(* Logix 5000 AddOnInstructionDefinition export Banner_Q90R2_KD_PD_v4; software revision 33.00 *)

TYPE Banner_Q90R2KD_PDI_0_v4 :   // Process Data for a Q90R2 sensors.
STRUCT
   SSC1_State : SINT;   // 0 = Inactive 1 = Active
   SSC1_Stability : SINT;   // 0 = No target or maginal, 1 = Valid.
   SSC2_State : SINT;   // 0 = Inactive 1 = Active
   SSC2_Stability : SINT;   // 0 = No target or maginal, 1 = Valid.
   SSC1_Distance : DINT;
   SSC1_Beam_Angle : DINT;
   SSC1_Velocity : DINT;
   SSC1_Signal_Strength : DINT;
   SSC2_Distance : DINT;
   SSC2_Beam_Angle : DINT;
   SSC2_Velocity : DINT;
   SSC2_Signal_Strength : DINT;
END_STRUCT
END_TYPE

TYPE Banner_Q90R2KD_PDI_1_v4 :   // Process Data for a Q90R2 sensors.
STRUCT
   SSC1_State : SINT;   // 0 = Inactive, 1 = True.
   SSC1_Stability : SINT;   // 0 = No target or maginal, 1 = Valid.
   SSC2_State : SINT;   // 0 = Inactive, 1 = True.
   SSC2_Stability : SINT;   // 0 = No target or maginal, 1 = Valid.
   SSC1_X : DINT;
   SSC1_Y : DINT;
   SSC1_Velocity : DINT;
   SSC1_Signal_Strength : DINT;
   SSC2_X : DINT;
   SSC2_Y : DINT;
   SSC2_Velocity : DINT;
   SSC2_Signal_Strength : DINT;
END_STRUCT
END_TYPE

TYPE Banner_Q90R2KD_PDI_v4 :   // Process Data for a Q90R2 sensors.
STRUCT
   Set_0 : Banner_Q90R2KD_PDI_0_v4;
   Set_1 : Banner_Q90R2KD_PDI_1_v4;
   PDI_DT : SINT[16];
END_STRUCT
END_TYPE

ADD_ON_INSTRUCTION Banner_Q90R2_KD_PD_v4   (* revision 4.0, vendor Banner Engineering *)
// Take raw process data and convert it to usable values.
VAR_IN_OUT
   PD : Banner_Q90R2KD_PDI_v4; {required}
END_VAR
VAR_INPUT
   PD_Layout : SINT; {required}
   Byte_Swap : BOOL; {required}
END_VAR
VAR
   Temp : SINT[16]; {access None}
END_VAR

ROUTINE Logic   (* ladder *)
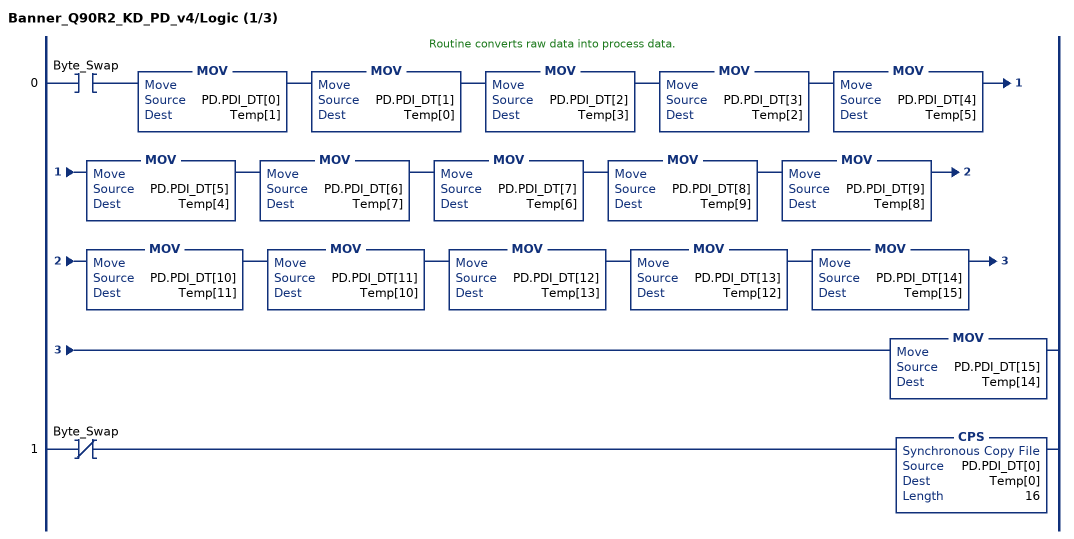
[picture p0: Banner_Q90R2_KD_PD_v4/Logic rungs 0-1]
   // Routine converts raw data into process data.
   0: XIC(Byte_Swap)MOV(PD.PDI_DT[0],Temp[1])MOV(PD.PDI_DT[1],Temp[0])MOV(PD.PDI_DT[2],Temp[3])MOV(PD.PDI_DT[3],Temp[2])MOV(PD.PDI_DT[4],Temp[5])MOV(PD.PDI_DT[5],Temp[4])MOV(PD.PDI_DT[6],Temp[7])MOV(PD.PDI_DT[7],Temp[6])MOV(PD.PDI_DT[8],Temp[9])MOV(PD.PDI_DT[9],Temp[8])MOV(PD.PDI_DT[10],Temp[11])MOV(PD.PDI_DT[11],Temp[10])MOV(PD.PDI_DT[12],Temp[13])MOV(PD.PDI_DT[13],Temp[12])MOV(PD.PDI_DT[14],Temp[15])MOV(PD.PDI_DT[15],Temp[14]);
   1: XIO(Byte_Swap)CPS(PD.PDI_DT[0],Temp[0],16);
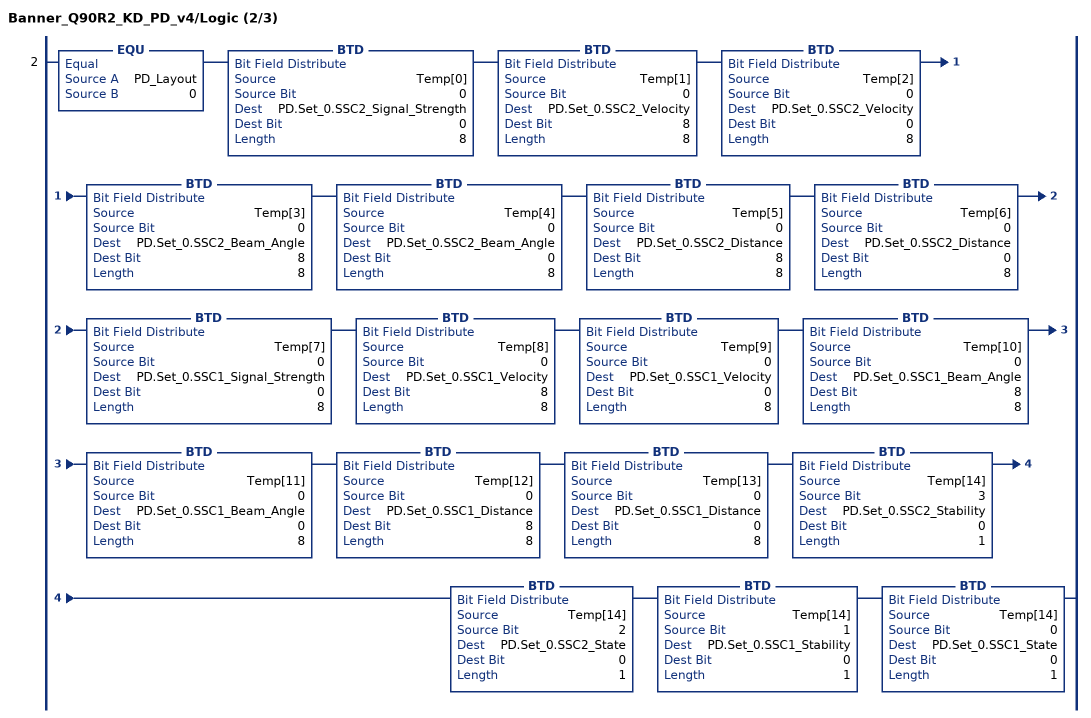
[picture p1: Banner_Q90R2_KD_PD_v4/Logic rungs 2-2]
   2: EQU(PD_Layout,0)BTD(Temp[0],0,PD.Set_0.SSC2_Signal_Strength,0,8)BTD(Temp[1],0,PD.Set_0.SSC2_Velocity,8,8)BTD(Temp[2],0,PD.Set_0.SSC2_Velocity,0,8)BTD(Temp[3],0,PD.Set_0.SSC2_Beam_Angle,8,8)BTD(Temp[4],0,PD.Set_0.SSC2_Beam_Angle,0,8)BTD(Temp[5],0,PD.Set_0.SSC2_Distance,8,8)BTD(Temp[6],0,PD.Set_0.SSC2_Distance,0,8)BTD(Temp[7],0,PD.Set_0.SSC1_Signal_Strength,0,8)BTD(Temp[8],0,PD.Set_0.SSC1_Velocity,8,8)BTD(Temp[9],0,PD.Set_0.SSC1_Velocity,0,8)BTD(Temp[10],0,PD.Set_0.SSC1_Beam_Angle,8,8)BTD(Temp[11],0,PD.Set_0.SSC1_Beam_Angle,0,8)BTD(Temp[12],0,PD.Set_0.SSC1_Distance,8,8)BTD(Temp[13],0,PD.Set_0.SSC1_Distance,0,8)BTD(Temp[14],3,PD.Set_0.SSC2_Stability,0,1)BTD(Temp[14],2,PD.Set_0.SSC2_State,0,1)BTD(Temp[14],1,PD.Set_0.SSC1_Stability,0,1)BTD(Temp[14],0,PD.Set_0.SSC1_State,0,1);
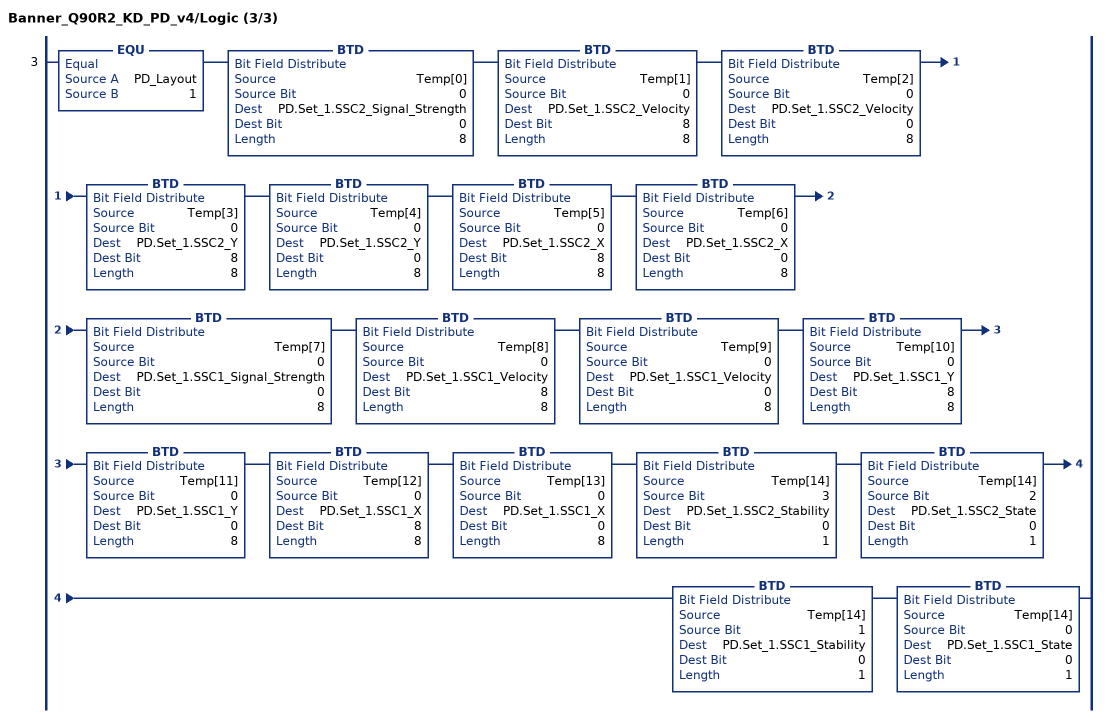
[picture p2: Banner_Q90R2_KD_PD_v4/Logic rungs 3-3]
   3: EQU(PD_Layout,1)BTD(Temp[0],0,PD.Set_1.SSC2_Signal_Strength,0,8)BTD(Temp[1],0,PD.Set_1.SSC2_Velocity,8,8)BTD(Temp[2],0,PD.Set_1.SSC2_Velocity,0,8)BTD(Temp[3],0,PD.Set_1.SSC2_Y,8,8)BTD(Temp[4],0,PD.Set_1.SSC2_Y,0,8)BTD(Temp[5],0,PD.Set_1.SSC2_X,8,8)BTD(Temp[6],0,PD.Set_1.SSC2_X,0,8)BTD(Temp[7],0,PD.Set_1.SSC1_Signal_Strength,0,8)BTD(Temp[8],0,PD.Set_1.SSC1_Velocity,8,8)BTD(Temp[9],0,PD.Set_1.SSC1_Velocity,0,8)BTD(Temp[10],0,PD.Set_1.SSC1_Y,8,8)BTD(Temp[11],0,PD.Set_1.SSC1_Y,0,8)BTD(Temp[12],0,PD.Set_1.SSC1_X,8,8)BTD(Temp[13],0,PD.Set_1.SSC1_X,0,8)BTD(Temp[14],3,PD.Set_1.SSC2_Stability,0,1)BTD(Temp[14],2,PD.Set_1.SSC2_State,0,1)BTD(Temp[14],1,PD.Set_1.SSC1_Stability,0,1)BTD(Temp[14],0,PD.Set_1.SSC1_State,0,1);
END_ROUTINE
END_ADD_ON_INSTRUCTION
